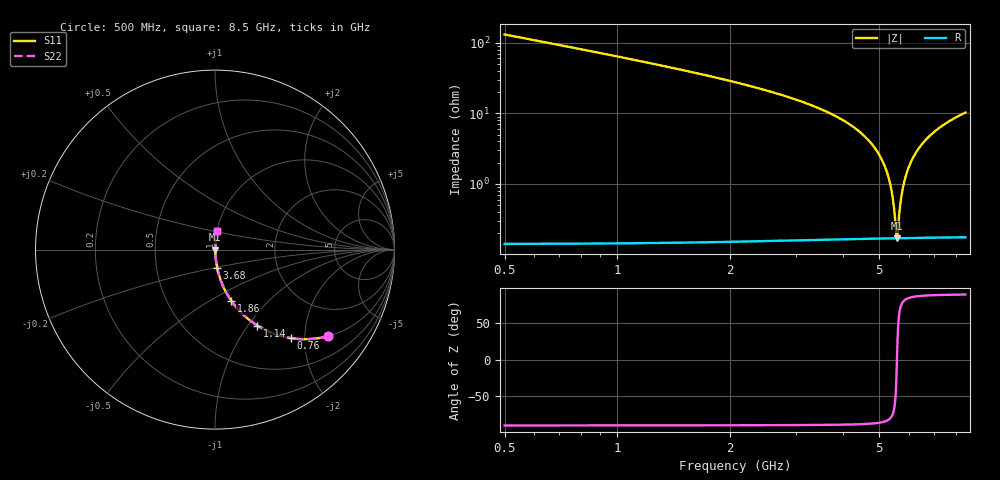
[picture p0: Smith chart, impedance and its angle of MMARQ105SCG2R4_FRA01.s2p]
! MMARQ105SCG2R4_FRA01  S-PARAMETER MODEL  ( General Type )
! Model Generated by TAIYO YUDEN Corporation (http://www.ty-top.com)
! Version 1.0
! TAIYO YUDEN Control No. 200326
! Copyright(c) 2020 TAIYO YUDEN CO.,LTD. All Rights Reserved.
! Product Description (link to TY-COMPAS)
! https://ds.yuden.co.jp/TYCOMPAS/or/detail?pn=MMARQ105SCG2R4BFRA01&u=M
! Products Name : Multilayer Ceramic Capacitors
! Characteristics :
!  Capacitance : 2.4 pF , Rated Voltage : 250V , TCC : CG / C0G
!  Case Size : 1.0 x 0.5 / 0.039 x 0.02 [mm/inch] , Thickness : 0.5 / 0.02 [mm/inch]
!  (Conditions: Temperature = 25 degC , DC Bias Current/Voltage = 0A / 0V)
! External Node Assignments :
!  1  o---| |---o  2
! GND o---------o GND
! Frequency Range : 500MHz  -  8.5GHz  [ 401 STEP ]
# MHz S RI R 50
! Freq[MHz].  S11 Real  S11 Imag  S21 Real  S21 Imag  S12 Real  S12 Imag  S22 Real  S22 Imag
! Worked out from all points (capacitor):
!   401 points, 500 MHz to 8.5 GHz, reference 50 ohm
!   read as one part in series: C = 2.41 pF near 540 MHz
!   lowest |Z| = 170 mohm at 5.58 GHz (marker M1)
!   series resonance near 5.58 GHz, so ESL is about 340 pH
!   S11 on the Smith chart (normalised r, x): 500 MHz: 1.00, -2.62; 760 MHz: 1.00, -1.71; 1.14 GHz: 1.00, -1.11; 1.86 GHz: 1.00, -0.63; 3.68 GHz: 1.00, -0.20; 8.5 GHz: 1.00, +0.21
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500  0.6323 -0.4816  0.3677 0.4816  0.3677 0.4816  0.6323 -0.4816
760  0.4218 -0.493  0.5782 0.493  0.5782 0.493  0.4218 -0.493
1140  0.2365 -0.4237  0.7635 0.4237  0.7635 0.4237  0.2365 -0.4237
1840  0.0941 -0.2896  0.9059 0.2896  0.9059 0.2896  0.0941 -0.2896
1860  0.0918 -0.2864  0.9082 0.2864  0.9082 0.2864  0.0918 -0.2864
3180  0.0208 -0.1372  0.9792 0.1372  0.9792 0.1372  0.0208 -0.1372
3680  0.0118 -0.1001  0.9882 0.1001  0.9882 0.1001  0.0118 -0.1001
4500  0.00428 -0.051  0.9957 0.051  0.9957 0.051  0.00428 -0.051
4940  0.00251 -0.0288  0.9975 0.0288  0.9975 0.0288  0.00251 -0.0288
5240  0.00191 -0.0148  0.9981 0.0148  0.9981 0.0148  0.00191 -0.0148
5420  0.00174 -0.00687  0.9983 0.00687  0.9983 0.00687  0.00174 -0.00687
5480  0.00171 -0.00427  0.9983 0.00427  0.9983 0.00427  0.00171 -0.00427
5540  0.0017 -0.0017  0.9983 0.0017  0.9983 0.0017  0.0017 -0.0017
5580  0.0017 -1.95e-06  0.9983 1.95e-06  0.9983 1.95e-06  0.0017 -1.95e-06
5620  0.0017 0.00168  0.9983 -0.00168  0.9983 -0.00168  0.0017 0.00168
5720  0.00174 0.00584  0.9983 -0.00584  0.9983 -0.00584  0.00174 0.00584
5840  0.00182 0.0107  0.9982 -0.0107  0.9982 -0.0107  0.00182 0.0107
6040  0.00206 0.0187  0.9979 -0.0187  0.9979 -0.0187  0.00206 0.0187
6320  0.00259 0.0294  0.9974 -0.0294  0.9974 -0.0294  0.00259 0.0294
6700  0.00361 0.0433  0.9964 -0.0433  0.9964 -0.0433  0.00361 0.0433
7180  0.00534 0.0599  0.9947 -0.0599  0.9947 -0.0599  0.00534 0.0599
8500  0.0121 0.1012  0.9879 -0.1012  0.9879 -0.1012  0.0121 0.1012
